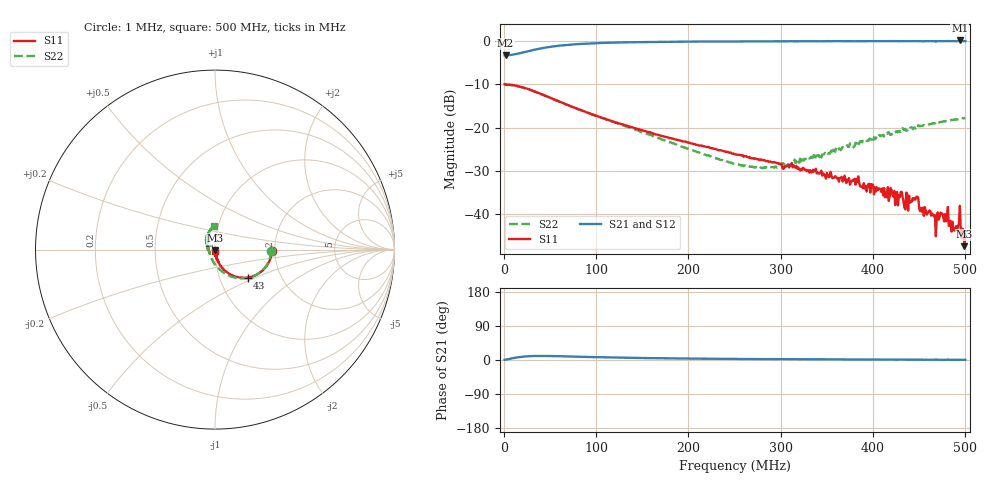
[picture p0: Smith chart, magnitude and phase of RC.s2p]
# Hz S RI R 50.0
! written by SimSmith version 18.3b
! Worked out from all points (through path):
!   500 points, 1 MHz to 500 MHz, reference 50 ohm
!   highest |S21| = 0.15 dB at 494 MHz (marker M1); lowest = -3.3 dB at 2 MHz (marker M2)
!   group delay of S21, straight-line fit = 51.9 ps
!   lowest |S11| = -47.4 dB at 499 MHz (marker M3), VSWR 1.01, Z = 50.2 - j0.38 ohm
!   |S11| at or under -10 dB: 2.79 MHz to end of sweep
!   |S22| runs from -29.4 to -10.1 dB; largest |S21 - S12| = 0
!   S11 on the Smith chart (normalised r, x): 1 MHz: 1.93, -0.03; 43 MHz: 1.36, -0.45; 500 MHz: 1.01, -0.01
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1000000  0.3171 -0.00687  0.6834 0.00625  0.6834 0.00625  0.3137 -0.00654
2000000  0.3163 -0.0123  0.6833 0.0122  0.6833 0.0122  0.3131 -0.0122
4.3e7  0.1811 -0.1554  0.8191 0.1561  0.8191 0.1561  0.1768 -0.1585
8.5e7  0.0806 -0.1356  0.9205 0.1357  0.9205 0.1357  0.0703 -0.141
1.68e8  0.0236 -0.0786  0.977 0.0788  0.977 0.0788  -0.00489 -0.0753
2.51e8  0.00976 -0.048  0.9909 0.0489  0.9909 0.0489  -0.0287 -0.0248
2.94e8  0.00658 -0.039  0.9938 0.0379  0.9938 0.0379  -0.0353 -0.00447
3.34e8  0.00488 -0.0302  0.9961 0.0325  0.9961 0.0325  -0.0421 0.0166
4.17e8  0.000977 -0.0143  0.9984 0.0194  0.9984 0.0194  -0.0477 0.0746
4.21e8  0.00393 -0.0163  0.9989 0.0165  0.9989 0.0165  -0.0431 0.0746
4.26e8  0.00843 -0.016  0.9989 0.0162  0.9989 0.0162  -0.0396 0.0788
4.3e8  0.000725 -0.018  0.9992 0.0176  0.9992 0.0176  -0.0414 0.0793
4.36e8  0.00639 -0.0166  0.998 0.0151  0.998 0.0151  -0.035 0.0853
4.47e8  0.00574 -0.0149  0.9978 0.0136  0.9978 0.0136  -0.0367 0.0946
4.53e8  0.00222 -0.0105  0.9979 0.0137  0.9979 0.0137  -0.0315 0.1006
4.66e8  0.00191 -0.0092  0.9979 0.0123  0.9979 0.0123  -0.0268 0.1094
4.74e8  0.00157 -0.01  0.9986 0.0109  0.9986 0.0109  -0.0221 0.1143
4.87e8  0.000455 -0.00652  0.9986 0.0112  0.9986 0.0112  -0.0149 0.1221
4.94e8  0.00484 -0.0115  1.017 0.00697  1.017 0.00697  -0.0051 0.1273
4.97e8  0.00289 -0.00614  0.9997 0.00886  0.9997 0.00886  -0.00551 0.1288
4.99e8  0.00199 -0.00378  0.9987 0.00895  0.9987 0.00895  -0.00567 0.129
5e8  0.00262 -0.00527  0.9988 0.00901  0.9988 0.00901  -0.00423 0.129
